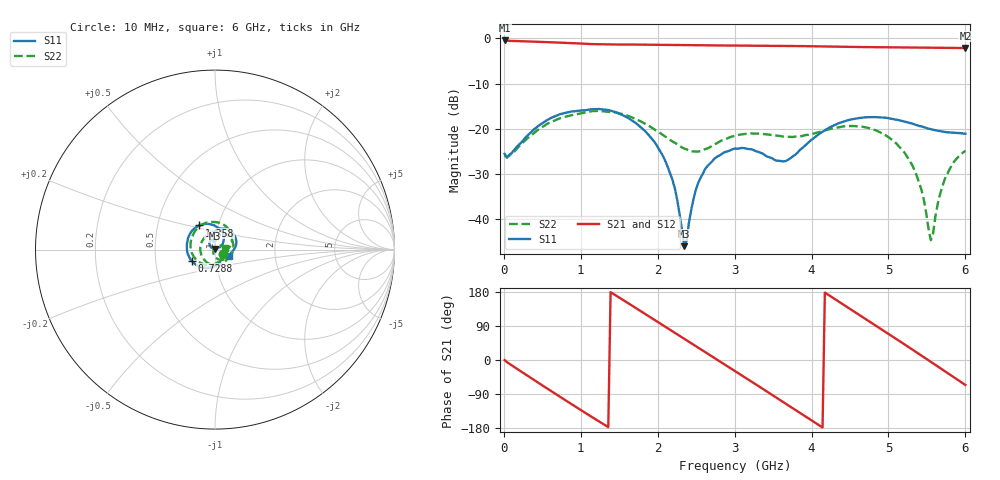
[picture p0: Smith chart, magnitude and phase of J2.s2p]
!Agilent Technologies,E8364B,MY43040528,A.07.50.67
!Agilent E8364B: A.07.50.67
!Date: Sunday, September 28, 2025 22:28:00
!Correction: S11(Full 2 Port(1,2))
!S21(Full 2 Port(1,2))
!S12(Full 2 Port(1,2))
!S22(Full 2 Port(1,2))
!S2P File: Measurements: S11, S21, S12, S22:
# Hz S  dB  R 50
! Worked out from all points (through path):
!   201 points, 10 MHz to 6 GHz, reference 50 ohm
!   highest |S21| = -0.44 dB at 10 MHz (marker M1); lowest = -2.1 dB at 6 GHz (marker M2)
!   group delay of S21, straight-line fit = 362 ps
!   lowest |S11| = -46.0 dB at 2.346 GHz (marker M3), VSWR 1.01, Z = 50.2 + j0.471 ohm
!   |S11| at or under -10 dB: start of sweep to end of sweep
!   |S22| runs from -44.7 to -16.1 dB; largest |S21 - S12| = 0.0073
!   S11 on the Smith chart (normalised r, x): 10 MHz: 1.09, -0.06; 728.8 MHz: 0.76, -0.10; 1.358 GHz: 0.81, +0.22; 6 GHz: 1.17, -0.09
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1e7  -25.56 -29.9  -0.44 -0.2  -0.48 0.1  -25.87 -31.2
3.9935e8  -20.02 -100.4  -0.71 -53.7  -0.71 -53.6  -20.84 -109.5
7.288e8  -16.79 -154.6  -0.93 -96.9  -0.92 -96.8  -17.68 -172.0
1.0283e9  -15.93 166.0  -1.15 -135.7  -1.15 -135.6  -16.49 141.2
1.35775e9  -15.85 123.5  -1.33 -177.2  -1.32 -177.1  -16.25 92.7
1.65725e9  -18.07 83.9  -1.35 144.7  -1.35 144.8  -17.40 53.3
2.01665e9  -24.54 40.5  -1.39 98.4  -1.40 98.4  -20.77 15.5
2.2263e9  -33.47 25.4  -1.45 71.3  -1.45 71.4  -23.13 3.0
2.3461e9  -45.99 69.4  -1.47 55.9  -1.47 56.1  -24.38 -0.8
2.49585e9  -33.48 151.5  -1.49 36.6  -1.49 36.7  -25.04 -0.3
2.61565e9  -28.95 143.0  -1.52 21.1  -1.51 21.2  -24.49 0.2
3.005e9  -24.36 109.6  -1.57 -29.2  -1.57 -29.0  -21.58 -34.0
3.27455e9  -24.95 90.3  -1.60 -64.2  -1.60 -64.1  -21.05 -74.3
3.51415e9  -26.85 88.4  -1.63 -95.4  -1.62 -95.3  -21.45 -117.8
4.0233e9  -22.12 104.3  -1.73 -162.3  -1.73 -162.2  -21.06 130.5
4.29285e9  -19.22 86.1  -1.81 162.2  -1.81 162.4  -19.82 76.8
4.59235e9  -17.69 61.2  -1.89 122.9  -1.89 123.0  -19.43 24.7
5.01165e9  -17.69 26.8  -1.96 67.5  -1.96 67.7  -21.99 -41.6
5.3411e9  -19.06 5.2  -2.00 23.5  -2.00 23.6  -29.26 -96.2
5.55075e9  -20.08 -4.1  -2.03 -4.8  -2.03 -4.6  -44.67 158.1
5.73045e9  -20.69 -10.0  -2.06 -29.2  -2.06 -29.0  -31.19 48.9
6e9  -21.08 -24.9  -2.12 -66.0  -2.12 -65.8  -24.88 8.3
